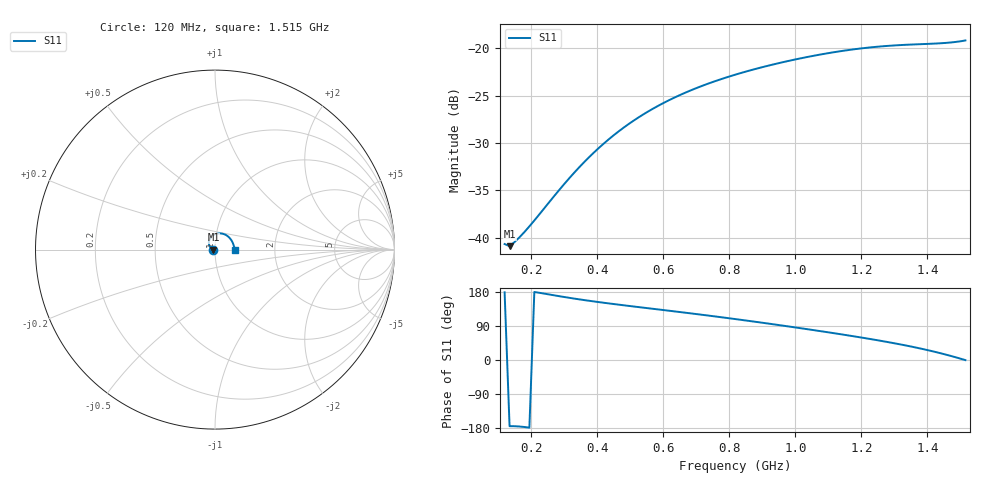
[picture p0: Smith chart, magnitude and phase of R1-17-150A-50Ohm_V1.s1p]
!version-1
!date-08.2020
!Series
#	GHZ S RI R 50.0
!	FREQ.GHZ	S11RE	S11IM
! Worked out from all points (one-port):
!   94 points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, 120 MHz to 1.515 GHz, reference 50 ohm
!   lowest |S11| = -40.9 dB at 135 MHz (marker M1), VSWR 1.02, Z = 49.1 - j0.0835 ohm
!   |S11| at or under -10 dB: start of sweep to end of sweep
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0.12  -0.00925 0.000217
0.135  -0.00897 -0.00085
0.15  -0.00943 -0.000871
0.165  -0.01 -0.000784
0.18  -0.0107 -0.000592
0.21  -0.0123 0.000104
0.3  -0.0186 0.00453
0.345  -0.022 0.00794
0.39  -0.0254 0.0121
0.435  -0.0284 0.0168
0.48  -0.0309 0.0221
0.51  -0.0323 0.0259
0.555  -0.0337 0.0319
0.6  -0.0342 0.0381
0.645  -0.0338 0.0446
0.69  -0.0324 0.0511
0.735  -0.0299 0.0576
0.825  -0.0216 0.0697
0.915  -0.00914 0.08
1.005  0.00714 0.0872
1.095  0.0264 0.09
1.17  0.0438 0.0879
1.26  0.0651 0.0787
1.35  0.0849 0.0608
1.41  0.0962 0.0432
1.455  0.1032 0.0265
1.485  0.1069 0.0137
1.515  0.1098 -0.000572
